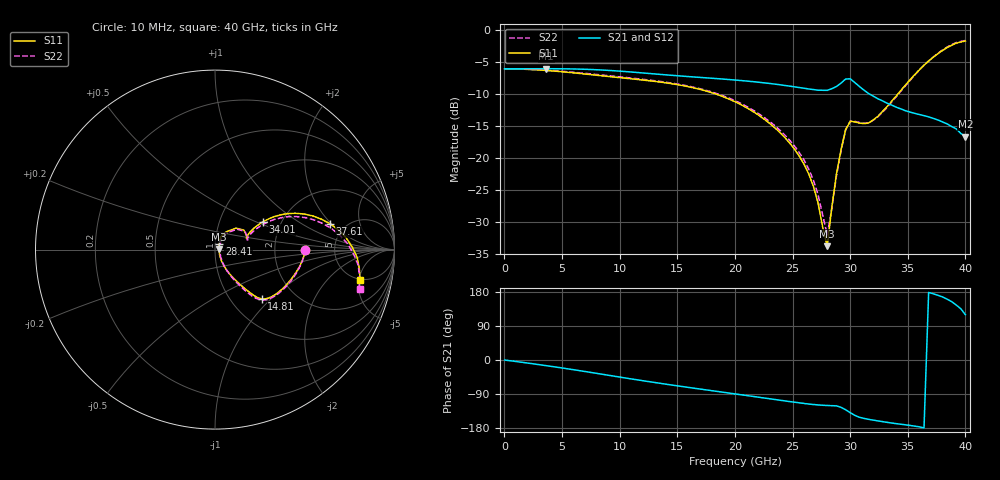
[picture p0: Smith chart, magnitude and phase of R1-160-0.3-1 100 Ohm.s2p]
!version-1
!date-09.2020
# MHz S RI R 50
!Freq ReS11 ImS11 ReS21 ImS21 ReS12 ImS12 ReS22 ImS22
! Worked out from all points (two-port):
!   101 points, 10 MHz to 40 GHz, reference 50 ohm
!   highest |S21| = -6.00 dB at 3.61 GHz (marker M1); lowest = -16.6 dB at 40 GHz (marker M2)
!   |S21| within 3 dB of the highest: start of sweep to 25.78 GHz; 28.56 GHz to 30.95 GHz (2.394 GHz wide, 8.05 % of centre)
!   lowest |S11| = -33.8 dB at 28.01 GHz (marker M3), VSWR 1.04, Z = 52 + j0.428 ohm
!   |S11| at or under -10 dB: 18.38 GHz to 34.12 GHz (15.74 GHz wide, 60 % of centre)
!   |S22| runs from -32.1 to -1.6 dB; largest |S21 - S12| = 0
!   S11 on the Smith chart (normalised r, x): 10 MHz: 3.00, -0.00; 14.81 GHz: 1.38, -0.88; 28.41 GHz: 1.05, +0.07; 34.01 GHz: 1.61, +0.55; 37.61 GHz: 3.80, +1.93; 40 GHz: 4.85, -5.18
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10  0.5001 -0.000183  0.4999 -0.000358  0.4999 -0.000358  0.5001 -0.000178
3610  0.4798 -0.076  0.4842 -0.1284  0.4842 -0.1284  0.4822 -0.075
6810  0.4283 -0.1599  0.4323 -0.2446  0.4323 -0.2446  0.4338 -0.1604
13610  0.2813 -0.2742  0.2121 -0.3987  0.2121 -0.3987  0.2814 -0.2804
14810  0.261 -0.274  0.1709 -0.4085  0.1709 -0.4085  0.2598 -0.2808
20010  0.1683 -0.2186  0.00345 -0.4086  0.00345 -0.4086  0.1666 -0.2266
24410  0.0716 -0.1228  -0.116 -0.3512  -0.116 -0.3512  0.0748 -0.1287
26010  0.0436 -0.0777  -0.1472 -0.32  -0.1472 -0.32  0.0481 -0.0831
26810  0.0324 -0.0506  -0.1586 -0.3055  -0.1586 -0.3055  0.0373 -0.0559
28010  0.02 0.00411  -0.1697 -0.2937  -0.1697 -0.2937  0.0249 -0.00116
28410  0.0241 0.0336  -0.1776 -0.301  -0.1776 -0.301  0.029 0.0283
28810  0.0307 0.0686  -0.1873 -0.3116  -0.1873 -0.3116  0.0355 0.0633
29210  0.0617 0.0987  -0.2215 -0.3167  -0.2215 -0.3167  0.0666 0.0934
29610  0.117 0.1195  -0.2756 -0.3121  -0.2756 -0.3121  0.1223 0.1137
30010  0.161 0.1084  -0.315 -0.2737  -0.315 -0.2737  0.1663 0.1019
31610  0.1756 0.0683  -0.2935 -0.1267  -0.2935 -0.1267  0.1792 0.0588
33610  0.2425 0.1389  -0.2525 -0.0617  -0.2525 -0.0617  0.2448 0.1262
34010  0.2657 0.1547  -0.2446 -0.0521  -0.2446 -0.0521  0.2679 0.1412
36010  0.4484 0.2024  -0.2188 -0.0135  -0.2188 -0.0135  0.4537 0.1839
37610  0.6413 0.1438  -0.1962 0.0318  -0.1962 0.0318  0.6509 0.116
38810  0.7647 0.0141  -0.1586 0.0775  -0.1586 0.0775  0.7729 -0.0257
40000  0.8083 -0.1697  -0.0726 0.1284  -0.0726 0.1284  0.8052 -0.2184
